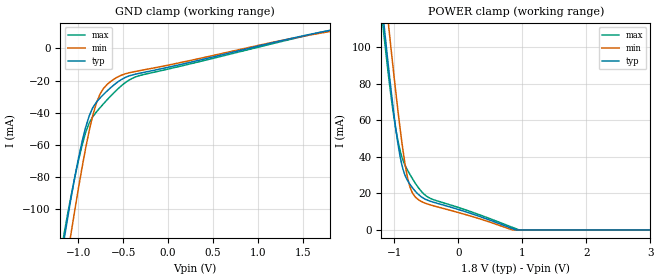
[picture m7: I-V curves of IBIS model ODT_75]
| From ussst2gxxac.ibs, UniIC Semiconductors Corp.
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|   Model ODT_75
[Model]  ODT_75
Model_type Input
Polarity   Non-Inverting
Vinl =   0.70000000V
Vinh =   1.10000000V
C_comp   2.5240pF   2.5060pF   2.5510pF
[Temperature Range]   25.0000   95.0000   0.0
[Voltage Range]   1.8000V   1.7000V   1.9000V
[GND_clamp]
|Voltage   I(typ)   I(min)   I(max)
-1.8V     -361.9mA   -386.3mA   -355mA
-1.16V    -119.4mA   -143mA     -115.6mA
-1.12V    -105.7mA   -128.6mA   -103.1mA
-1.08V    -92.48mA   -114.5mA   -91.32mA
-960mV    -58.29mA   -74.42mA   -60.54mA
-880mV    -42.09mA   -51.33mA   -46.48mA
-840mV    -36.92mA   -41.77mA   -42.53mA
-760mV    -30.94mA   -28.54mA   -36.97mA
-600mV    -22.54mA   -18.99mA   -27.33mA
-440mV    -17.21mA   -15.24mA   -19.86mA
-320mV    -15.47mA   -13.85mA   -16.94mA
1.8V      11.22mA    10.51mA    11.17mA
[POWER_clamp]
|Voltage   I(typ)   I(min)   I(max)
-1.8V     342.3mA    366.4mA    335mA
-1.18V    119.6mA    143.7mA    113.5mA
-1.16V    112.9mA    136.8mA    106.9mA
-1.14V    106.2mA    129.9mA    100.5mA
-1.08V    86.57mA    109.7mA    82.08mA
-940mV    47.02mA    65.1mA     48.76mA
-820mV    29.07mA    34.09mA    34.64mA
-740mV    24.29mA    22.29mA    29.54mA
-600mV    18.78mA    16.08mA    22.14mA
-400mV    15.31mA    13.35mA    16.74mA
903.9mV   0A         NA         NA
3.6V      0A         0A         0A
